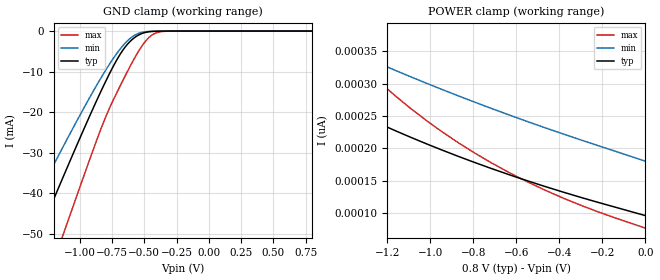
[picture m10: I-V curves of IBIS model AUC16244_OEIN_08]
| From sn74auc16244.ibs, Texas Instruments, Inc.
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[Model]   AUC16244_OEIN_08
Model_type  Input
Vinl=0
Vinh=0.8
| variable   typ   min   max
C_comp   2.61pF   2.27pF   2.93pF
[Temperature Range]   40   100   -40
| Ambient temperature   25   85   -40
[Voltage range]   0.8   0.8   0.8
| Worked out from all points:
|   GND clamp passes 1 mA (typ) near -0.55 V on its own axis
[GND Clamp]
| AUC16244_OEIN_08
|   Voltage   I(typ)   I(min)   I(max)
-3.6V     -226.6mA   -190.3mA   -271.8mA
-1.485V   -63.01mA   -50.7mA    -82.58mA
-1.445V   -59.95mA   -48.16mA   -78.96mA
-1.305V   -49.28mA   -39.36mA   -66.26mA
-1.135V   -36.48mA   -28.9mA    -50.82mA
-1.1V     -33.88mA   -26.79mA   -47.64mA
-840mV    -15.17mA   -11.81mA   -24.5mA
-695mV    -6.152mA   -4.773mA   -14.06mA
-580mV    -1.726mA   -1.13mA    -6.949mA
-450mV    -123.7uA   -59.61uA   -1.212mA
-315mV    -2.431uA   -1.534uA   -21.15uA
800mV     96.17pA    180.2pA    76.88pA
[POWER Clamp]
| AUC16244_OEIN_08
|   Voltage   I(typ)   I(min)   I(max)
-3.6V     886.1pA    812.4pA    2.692nA
-2.02V    380.6pA    456.8pA    643.3pA
-1.555V   290pA      379pA      413.6pA
-1.495V   279.7pA    369.7pA    390.3pA
-1.43V    268.9pA    359.7pA    366.4pA
-1.295V   247.4pA    339.7pA    321pA
-1.09V    217.2pA    310.7pA    261.7pA
-945mV    197.5pA    291.2pA    225.8pA
-795mV    178.5pA    271.8pA    193.3pA
-470mV    141.6pA    232.4pA    136.1pA
-215mV    116.2pA    203.8pA    101.4pA
-54.69fV  96.17pA    180.2pA    76.88pA
